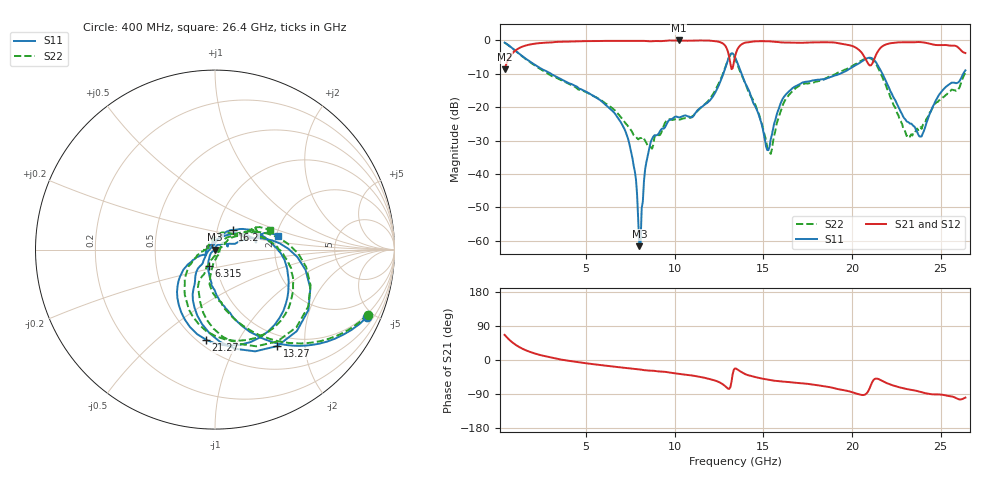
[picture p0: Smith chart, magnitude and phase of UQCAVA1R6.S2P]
!  Part Number  UQCAVA1R6
!  Description: RF capacitor  Mounting Orientation: Horizontal
!  Application:
# GHZ S DB R 50
! Freq  |S11|  S11 Ph  |S21|  S21 Ph  |S12|  S12 Ph  |S22|  S22 Ph
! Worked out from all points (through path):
!   401 points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, 400 MHz to 26.4 GHz, reference 50 ohm
!   highest |S21| = 0.00 dB at 10.21 GHz (marker M1); lowest = -8.6 dB at 400 MHz (marker M2)
!   group delay of S21, straight-line fit = 12.7 ps
!   lowest |S11| = -61.6 dB at 8.005 GHz (marker M3), VSWR 1.00, Z = 50 - j0.0832 ohm
!   |S11| at or under -10 dB: 3.026 GHz to 12.74 GHz (9.713 GHz wide, 123 % of centre); 13.78 GHz to 19.32 GHz (5.548 GHz wide, 33.5 % of centre); 21.72 GHz to 26.28 GHz (4.555 GHz wide, 19 % of centre)
!   |S22| runs from -34.0 to -0.7 dB; largest |S21 - S12| = 0.0089
!   S11 on the Smith chart (normalised r, x): 400 MHz: 0.87, -4.59; 6.315 GHz: 0.92, -0.17; 13.27 GHz: 0.83, -1.50; 16.2 GHz: 1.19, +0.26; 21.27 GHz: 0.55, -0.74; 26.4 GHz: 2.03, +0.36
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0.4  -0.66 -23.8  -8.60 66.3  -8.63 66.3  -0.68 -23.0
1.895  -6.57 -69.1  -1.14 20.4  -1.17 20.5  -6.72 -68.9
4.755  -14.70 -96.3  -0.21 -7.1  -0.23 -6.9  -14.91 -98.0
6.315  -20.29 -111.9  -0.13 -16.1  -0.13 -15.8  -19.66 -98.5
7.42  -30.51 -139.3  -0.14 -22.0  -0.13 -21.7  -25.98 -83.0
8.005  -61.60 -91.2  -0.14 -24.9  -0.12 -24.5  -29.33 -45.5
8.525  -33.22 69.1  -0.23 -27.9  -0.21 -27.5  -31.79 -19.1
9.11  -27.76 42.9  -0.21 -30.1  -0.19 -29.8  -28.39 24.2
10.215  -23.02 19.9  0.00 -36.7  -0.01 -36.4  -23.66 33.8
12.685  -10.81 11.9  -0.81 -63.2  -0.79 -63.1  -10.43 17.4
13.27  -3.88 -57.1  -8.30 -37.0  -8.28 -37.0  -4.17 -55.8
13.4  -4.97 -78.4  -4.85 -22.3  -4.83 -22.3  -5.38 -76.7
13.79  -10.20 -113.5  -1.11 -32.6  -1.09 -32.5  -10.62 -106.7
15.22  -32.81 144.8  -0.24 -51.6  -0.20 -51.6  -32.09 -76.1
16.195  -16.66 47.8  -0.62 -57.2  -0.60 -57.3  -18.20 34.6
17.755  -12.00 21.1  -0.59 -64.6  -0.55 -64.8  -12.60 25.9
20.485  -6.53 -30.1  -3.28 -91.7  -3.23 -91.9  -6.19 -27.4
21.265  -5.93 -95.6  -5.46 -50.5  -5.42 -50.8  -6.35 -89.7
22.11  -14.43 -149.3  -0.91 -63.7  -0.88 -64.0  -16.09 -149.0
23.15  -24.39 -152.7  -0.55 -77.2  -0.52 -77.6  -28.14 172.9
23.865  -28.77 135.7  -0.49 -84.2  -0.46 -84.6  -25.93 116.7
26.4  -8.95 12.6  -3.77 -99.3  -3.74 -99.8  -9.71 19.3
